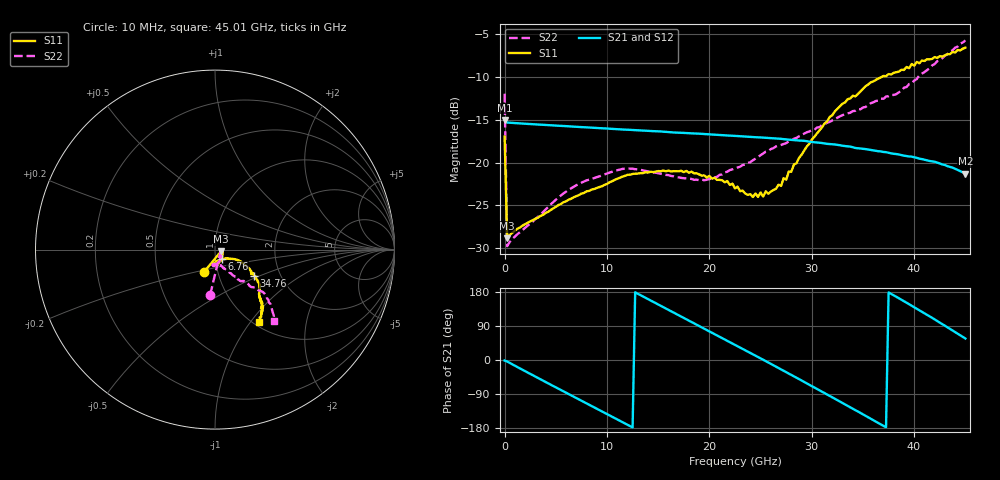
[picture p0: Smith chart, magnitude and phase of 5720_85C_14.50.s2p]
! Device:  ADRF5720
! Description: 0.5dB LSB GaAs MMIC 6-bit Digital Attenuator
! Frequency:  0.000009 -  40 GHz
! Ports:
!	RF1	= Port 1
!	RF2	= Port 2
! Vdd:  3.3 Volt
! Vss:  -3.3 Volt
! Control:  0/3.3 Volt
! State:  14.50 dB attenuation
! Data:  The device was measured using G-S-G Probes on a matrix board.
!  Data was collected using an calibrated 4 port network analyzer.
!  The reference plane for this measurement is at the launchers.
! Note:  Analog Devices supplies this data as a sample of measured data
!  for this product.  Your particular data for this product may vary.
!  Data was taken at 85 degrees C.
!  Analog Devices reserves the right to change this data at anytime.
# GHZ S DB R 45.0
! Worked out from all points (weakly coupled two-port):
!   181 points, 10 MHz to 45.01 GHz, reference 45 ohm
!   highest |S21| = -15.03 dB at 10 MHz (marker M1); lowest = -21.3 dB at 45.01 GHz (marker M2)
!   lowest |S11| = -28.9 dB at 260 MHz (marker M3), VSWR 1.07, Z = 48.3 - j0.822 ohm
!   |S11| at or under -10 dB: start of sweep to 36.83 GHz
!   |S22| runs from -29.8 to -5.7 dB; largest |S21 - S12| = 0.00087
!   S11 on the Smith chart (normalised r, x): 10 MHz: 0.85, -0.22; 6.76 GHz: 1.07, -0.11; 34.76 GHz: 1.47, -0.45; 45.01 GHz: 1.06, -1.09
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0.01  -16.96 -116.5  -15.03 -1.4  -15.02 -1.4  -11.96 -96.1
0.26  -28.85 -13.6  -15.33 -4.0  -15.33 -4.0  -29.78 -15.1
3.76  -26.13 -31.9  -15.59 -54.5  -15.58 -54.4  -25.81 -46.6
6.76  -24.06 -54.1  -15.80 -96.9  -15.79 -96.9  -22.83 -71.6
7.76  -23.56 -59.6  -15.87 -111.0  -15.86 -111.0  -22.22 -77.0
11.76  -21.56 -78.8  -16.15 -167.3  -16.14 -167.2  -20.73 -94.2
15.26  -21.02 -90.1  -16.37 143.1  -16.36 143.3  -21.31 -99.6
19.01  -21.40 -94.6  -16.63 90.1  -16.62 90.2  -22.06 -88.5
22.76  -22.82 -85.6  -16.91 36.6  -16.89 36.8  -20.59 -71.5
24.76  -24.02 -70.9  -17.05 7.9  -17.04 8.2  -19.35 -66.3
27.01  -22.73 -43.0  -17.23 -24.8  -17.22 -24.6  -17.94 -60.5
27.26  -21.83 -39.4  -17.27 -28.5  -17.25 -28.3  -17.82 -60.7
27.51  -22.01 -37.8  -17.30 -32.1  -17.28 -31.9  -17.73 -59.5
27.76  -21.06 -34.5  -17.32 -35.8  -17.31 -35.5  -17.51 -60.0
28.01  -21.08 -34.5  -17.35 -39.5  -17.34 -39.2  -17.42 -59.1
30.26  -16.99 -26.3  -17.63 -72.5  -17.61 -72.2  -16.18 -56.8
33.01  -13.12 -29.0  -18.04 -113.6  -18.03 -113.3  -14.46 -53.6
34.76  -11.70 -33.7  -18.35 -139.7  -18.33 -139.4  -13.78 -52.6
37.76  -9.71 -40.8  -18.93 174.5  -18.91 174.9  -12.10 -46.8
41.51  -7.93 -49.7  -19.82 115.3  -19.79 115.7  -8.99 -41.5
43.51  -7.33 -52.0  -20.51 82.2  -20.48 82.6  -7.02 -45.5
45.01  -6.57 -58.9  -21.29 56.7  -21.26 57.0  -5.73 -50.5
